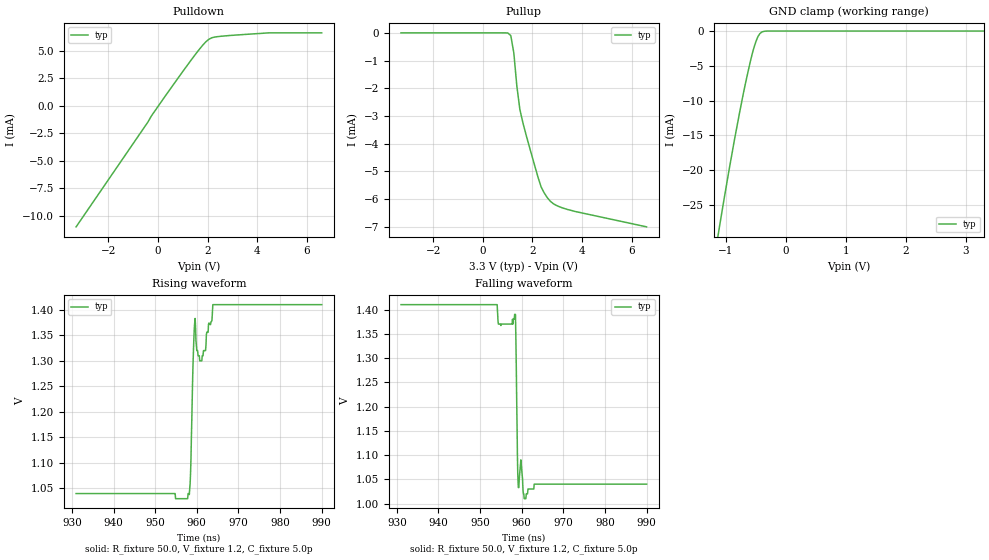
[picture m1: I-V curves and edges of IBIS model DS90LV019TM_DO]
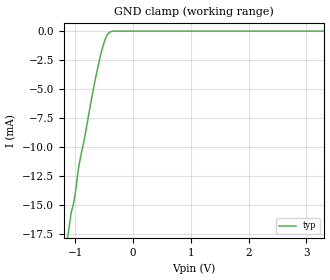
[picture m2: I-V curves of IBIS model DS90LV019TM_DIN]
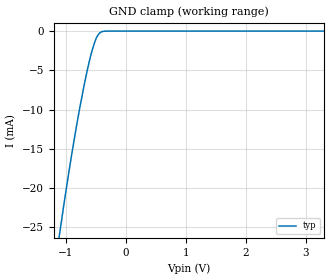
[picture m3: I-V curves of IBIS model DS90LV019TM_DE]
|   National Semiconductor Corporation
|   Interface Products Group
|   IBIS Model of DS90LV019TM
|   14L SOIC Package
[IBIS Ver]   2.1
[File name]   lv019tm.ibs
[Date]   03/08/02
[File Rev]   1.1
[Source]   Model Originated at National Semiconductor.
[Notes]   File created by BM from empirical data and
   verified by BM & SBH.
   File rev 1.1  fixes monotonicity and R_fixture
   Reason is to remove all warnings and any errors
   reported by ibischk3-----milt
   Checked with ibischk3 ver 3.2.5 on 3/8/2002----OK milt
[Disclaimer]
(C) Copyright National Semiconductor Corporation 1994
   All rights reserved
   National Semiconductor Corporation hereby grants
the user of this IBIS model a non-exclusive, nontransferable
license to use this IBIS model under the following terms.
Before using this IBIS model, the user should read this
license.  If the user does not accept these terms,  the
IBIS model should be returned to National within 30 days.
   The user is granted this license only to use the
IBIS model and is not granted rights to sell, load, rent,
lease or license the IBIS model in whole or in part, or in
modified form to anyone other than user. User may modify
the IBIS model to suit its specific applications but rights
to derivative works and such modifications shall belong to
National.
   This IBIS model is provided on an "AS IS" basis and
National makes absolutely no warranty with respect to the
information contained herein.NATIONAL DISCLAIMS AND CUSTOMER
WAIVES ALL WARRANTIES, EXPRESS OR IMPLIED, INCLUDING
WARRANTIES OF MERCHANTABILITY OR FITNESS FOR A PARTICULAR
PURPOSE. The entire risk as to quality and performance is
with the Customer. ACCORDINGLY, IN NO EVENT SHALL THE
COMPANY BE LIABLE FOR ANY DAMAGES, WHETHER IN CONTRACT OR
TORT,INCLUDING ANY LOST PROFITS OR OTHER INCIDENTAL,
CONSEQUENTIAL, EXEMPLARY, OR PUNITIVE DAMAGES ASING OUT
OF THE USE OR APPLICATION OF THE IBIS model provided in
this package.Further, National reserves the right to make
changes without notice to any product herein to improve
reliability, function, or design. National does not convey
any license under patent rights or any other intellectual
property rights, including those of third parties.
   National is not obligated to provide maintenance or support
for the licensed IBIS model.
Contact National at ATTN:INTERFACE APPLICATIONS/IBIS MODELS.
2900 Semiconductor Drive, M/S A2595, Santa Clara, CA 95052-8090
|   COMPONENT: DS90LV019TM
[Component]   DS90LV019TM
[Manufacturer]  National Semiconductor Corporation
[Package]
| variable   typ   min   max
R_pkg   50m   25m   75m
L_pkg   1.47n   1.05n   2.11n
C_pkg   0.28p   0.16p   0.40p
[Pin]   signal_name   model_name   R_pin   L_pin   C_pin
  1   DE   DS90LV019TM_DE   50m   2.11366n   0.40067p
  2   DIN   DS90LV019TM_DIN   50m   1.64135n   0.37335p
  3   NC   NC   50m   1.05193n   0.16890p
  4   ROUT   DS90LV019TM_ROUT   50m   1.05308n   0.16861p
  5   NC   NC   50m   1.05193n   0.16890p
  6   NC   NC   50m   1.64135n   0.37335p
  7   GND   GND   50m   2.11367n   0.40067p
  8   RE*   DS90LV019TM_RE   50m   2.11367n   0.40067p
  9   RI-   DS90LV019TM_RI   50m   1.64135n   0.37335p
  10   RI+   DS90LV019TM_RI   50m   1.05193n   0.16890p
  11   DO-   DS90LV019TM_DO   50m   1.05308n   0.16861p
  12   DO+   DS90LV019TM_DO   50m   1.05193n   0.16890p
  13   NC   NC   50m   1.64135n   0.37335p
  14   VCC   POWER   50m   2.11366n   0.40067p
[Diff_pin]   inv_pin   vdiff   tdelay_typ   tdelay_min   tdelay_max
| The '+' pin is Diff_pin and the '-' pin is the inv_pin
10   9   0.1   0 0 0
| Models and submodels in the file (6): DS90LV019TM_DO (3-state), DS90LV019TM_DIN (Input), DS90LV019TM_DE (Input), DS90LV019TM_RE (Input), DS90LV019TM_RI (Input), DS90LV019TM_ROUT (3-state)
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|   Driver Output MODEL {START}
[Model]   DS90LV019TM_DO
Model_type   3-state
|Signals   DO-,DO+
Vmeas = 1.2V   |Reference voltage for timing measurements
Cref = 5pF   |Timing specification test load capacitance value
Rref = 50   |Note: 100 Ohm between the two driver outputs
Vref = 1.2   |Timing specification test load voltage; GND
|   typ   min   max
C_comp   4.13pF   NA   NA
|   typ   min   max
[Temperature Range]   25.0   NA   NA
[Voltage range]   3.3V   3.0V   3.6V
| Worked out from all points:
|   slope of the pulldown table from 0 to 0.495 V, typ, clamps not added: 312 ohm
|   GND clamp passes 1 mA (typ) near -0.47 V on its own axis
|   rising waveform, R_fixture 50.0, V_fixture 1.2, C_fixture 5.0p: 20-80 % time 650ps typ, NA min, NA max; typ from 1.04 V to 1.41 V
|   falling waveform, R_fixture 50.0, V_fixture 1.2, C_fixture 5.0p: 20-80 % time 343ps typ, NA min, NA max; typ from 1.41 V to 1.04 V
[Pulldown]
|Voltage   I(typ)   I(min)   I(max)
-3.3V     -11.01mA   NA         NA
337mV     998uA      NA         NA
1.562V    4.801mA    NA         NA
1.807V    5.488mA    NA         NA
2.053V    6.021mA    NA         NA
2.175V    6.158mA    NA         NA
2.541V    6.294mA    NA         NA
4.378V    6.589mA    NA         NA
6.6V      6.605mA    NA         NA
[Pullup]
|Voltage   I(typ)   I(min)   I(max)
| Note that the[Pullup]voltage table is referenced to Vcc
| and is calculated using Vtable=Vcc - Vmeasured.
-3.3V     1.572uA    NA         NA
1.003V    -3.145uA   NA         NA
1.126V    -98.02uA   NA         NA
1.248V    -722.3uA   NA         NA
1.37V     -1.921mA   NA         NA
1.493V    -2.773mA   NA         NA
1.615V    -3.251mA   NA         NA
2.35V     -5.571mA   NA         NA
2.595V    -5.952mA   NA         NA
2.84V     -6.173mA   NA         NA
3.453V    -6.392mA   NA         NA
6.6V      -7.01mA    NA         NA
[Power_clamp]
| Note that the[POWER_clamp]voltage table is referenced to Vcc
| and is calculated using Vtable=Vcc - Vmeasured.
| Voltage   I(typ)   I(min)   I(max)
-3.3V     0A         NA         NA
0V        0A         NA         NA
[GND_clamp]
|Voltage   I(typ)   I(min)   I(max)
-3.3V     -151mA     NA         NA
-1.133V   -29.74mA   NA         NA
-1.103V   -28.12mA   NA         NA
-950mV    -20.3mA    NA         NA
-858mV    -15.85mA   NA         NA
-766mV    -11.64mA   NA         NA
-643mV    -6.466mA   NA         NA
-582mV    -4.15mA    NA         NA
-521mV    -2.174mA   NA         NA
-460mV    -771.3uA   NA         NA
-398mV    -147.8uA   NA         NA
3.3V      0A         NA         NA
[Ramp]
|   typ   min   max
dV/dt_r   0.209/0.790ns   NA   NA
dV/dt_f   0.207/0.709ns   NA   NA
R_load = 100Ohm
|D019opr
[Rising Waveform]
R_fixture = 50.0
V_fixture = 1.2
C_fixture = 5.0p | Jig capacitance
|  Time   V(Typ)   V(Min)   V(Max)
931ns     1.04V      NA         NA
957.8ns   1.03V      NA         NA
958.4ns   1.06V      NA         NA
959.1ns   1.283V     NA         NA
959.6ns   1.383V     NA         NA
960ns     1.32V      NA         NA
961.2ns   1.3V       NA         NA
963.6ns   1.379V     NA         NA
963.9ns   1.41V      NA         NA
990ns     1.41V      NA         NA
|D019opf
[Falling Waveform]
R_fixture = 50.0
V_fixture = 1.2
C_fixture = 5.0p | Jig capacitance
|   Time   V(Typ)   V(Min)   V(Max)
931ns     1.41V      NA         NA
954.1ns   1.41V      NA         NA
955ns     1.367V     NA         NA
958.5ns   1.39V      NA         NA
959ns     1.1V       NA         NA
959.2ns   1.033V     NA         NA
959.8ns   1.09V      NA         NA
960.6ns   1.01V      NA         NA
963ns     1.04V      NA         NA
990ns     1.04V      NA         NA
|   Driver Input MODEL {START}
[Model]   DS90LV019TM_DIN
Model_type   Input
|Signals   DIN
Vinh = 2.0
Vinl = 0.8
|   typ   min   max
C_comp   2.50pF   NA   NA
|   typ   min   max
[Temperature Range]   25.0   NA   NA
[Voltage range]   3.3V   3.0V   3.6V
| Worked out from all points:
|   GND clamp passes 1 mA (typ) near -0.50 V on its own axis
[Power_clamp]
| Note that the[POWER_clamp]voltage table is referenced to Vcc
| and is calculated using Vtable=Vcc - Vmeasured.
|   Voltage   I(typ)   I(min)   I(max)
-3.3V     0A         NA         NA
0V        0A         NA         NA
[GND_clamp]
|Voltage   I(typ)   I(min)   I(max)
-3.3V     -150mA     NA         NA
-1.133V   -17.7mA    NA         NA
-1.103V   -16.7mA    NA         NA
-1.072V   -15.59mA   NA         NA
-1.011V   -14.28mA   NA         NA
-950mV    -11.94mA   NA         NA
-919mV    -11.06mA   NA         NA
-644mV    -3.878mA   NA         NA
-552mV    -1.816mA   NA         NA
-490mV    -780uA     NA         NA
-399mV    -79.67uA   NA         NA
3.3V      157.2nA    NA         NA
|   Driver Enable MODEL {START}
[Model]   DS90LV019TM_DE
Model_type   Input
|Signals   DE
Vinh = 2.0
Vinl = 0.8
|   typ   min   max
C_comp   2.95pF   NA   NA
|   typ   min   max
[Temperature Range]   25.0   NA   NA
[Voltage range]   3.3V   3.0V   3.6V
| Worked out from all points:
|   GND clamp passes 1 mA (typ) near -0.50 V on its own axis
[GND_clamp]
|Voltage   I(typ)   I(min)   I(max)
-3.3V     -150mA     NA         NA
-1.103V   -25.78mA   NA         NA
-1.072V   -24.19mA   NA         NA
-950mV    -18.01mA   NA         NA
-827mV    -12.32mA   NA         NA
-705mV    -7.277mA   NA         NA
-644mV    -5.037mA   NA         NA
-583mV    -3.056mA   NA         NA
-521mV    -1.466mA   NA         NA
-460mV    -452.4uA   NA         NA
-399mV    -74.96uA   NA         NA
3.3V      304.1nA    NA         NA
[Power_clamp]
| Note that the[POWER_clamp]voltage table is referenced to Vcc
| and is calculated using Vtable=Vcc - Vmeasured.
|   Voltage   I(typ)   I(min)   I(max)
-3.3V     0A         NA         NA
0V        0A         NA         NA
